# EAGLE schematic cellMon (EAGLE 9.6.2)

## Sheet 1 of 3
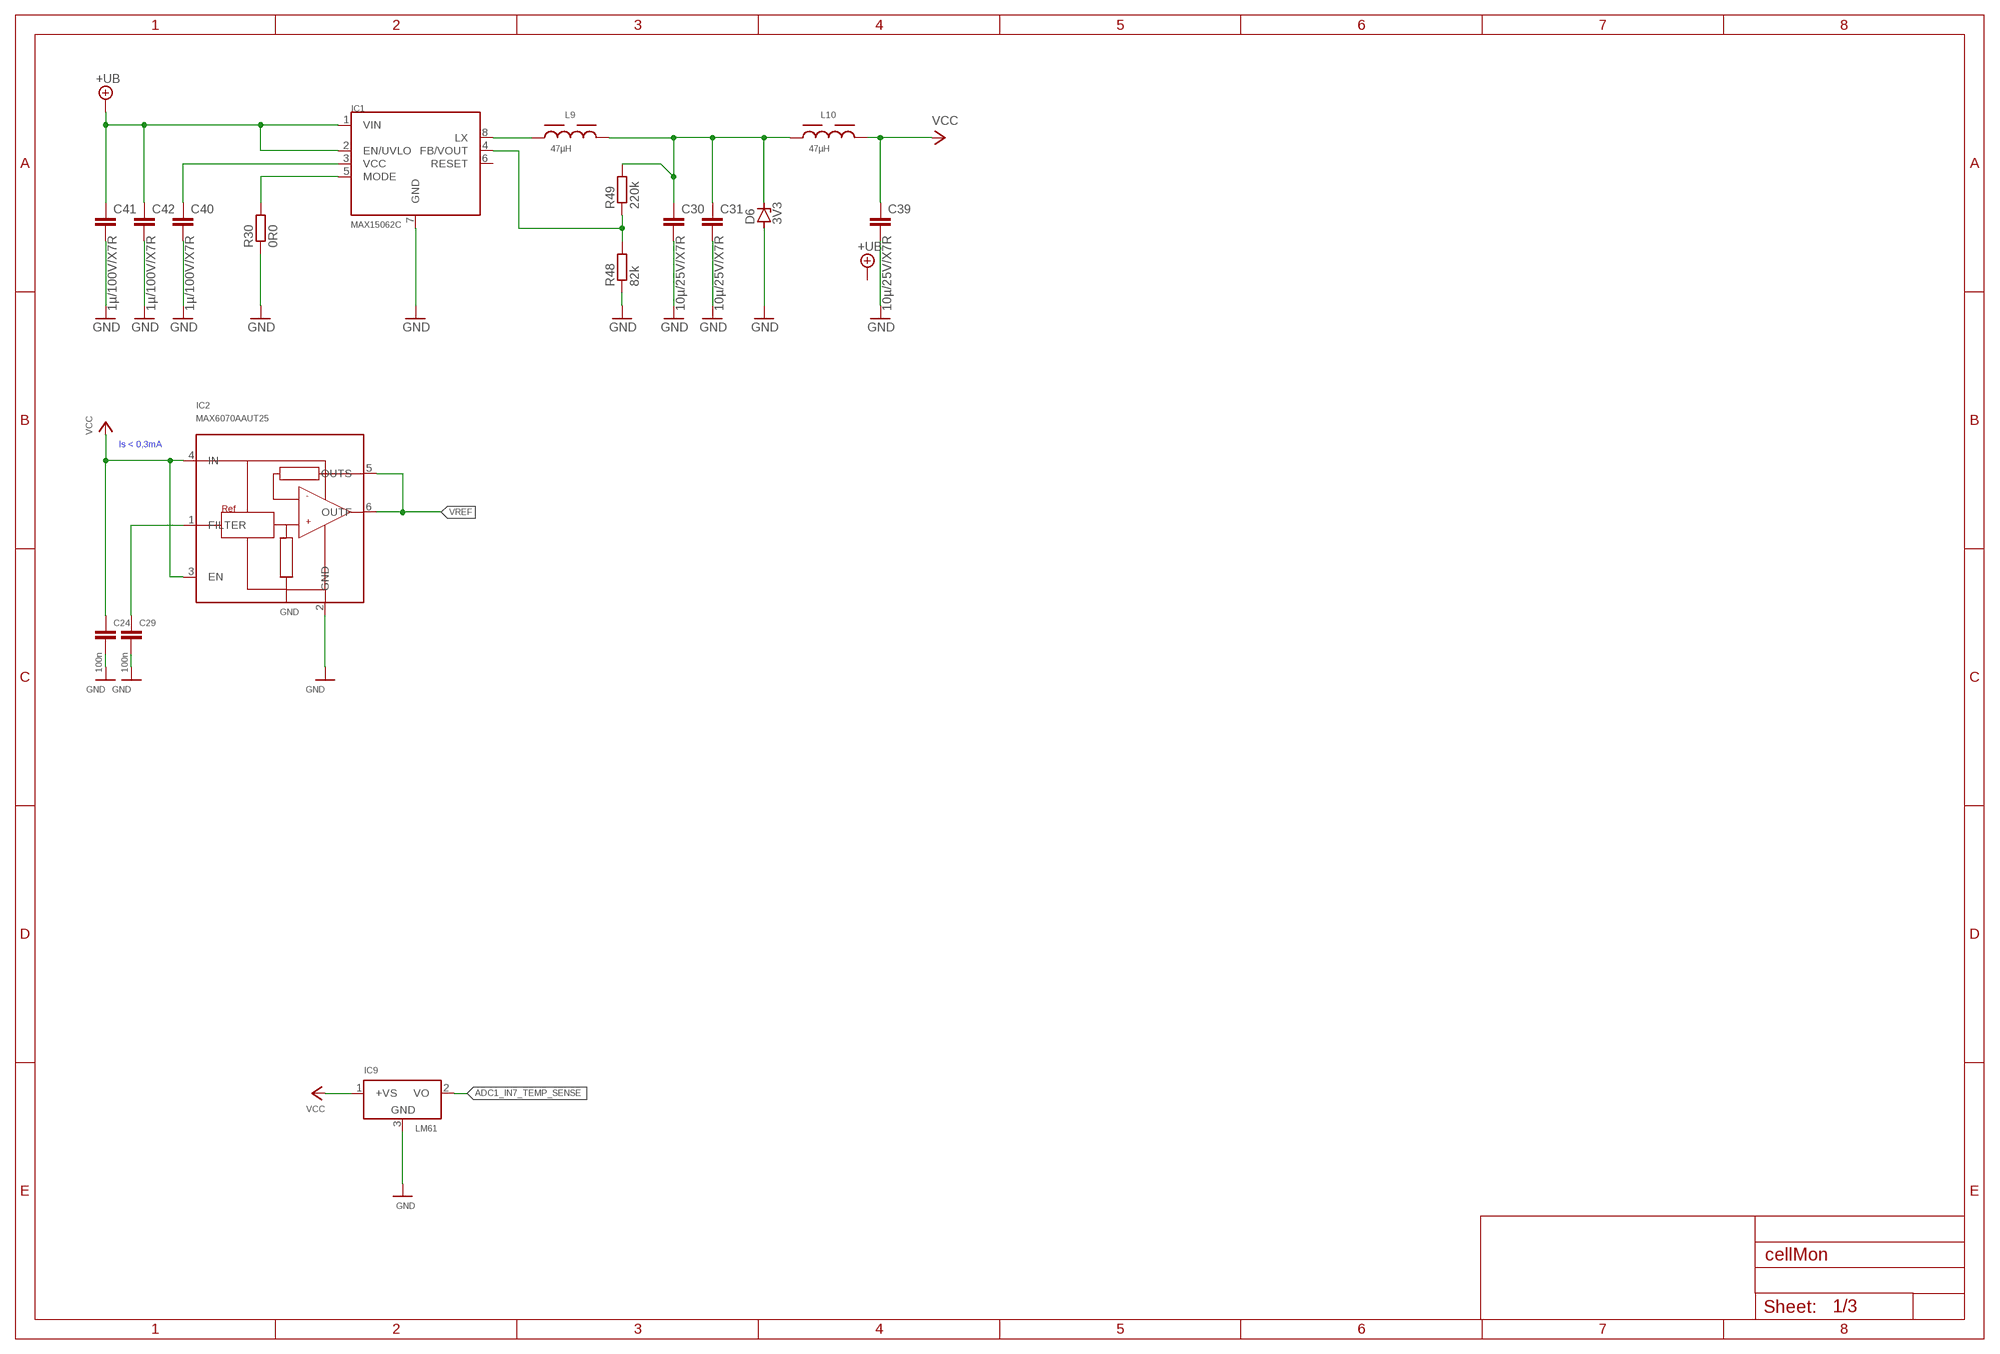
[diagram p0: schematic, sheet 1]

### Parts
C24  100n  C-EUC0603K  [C0603K]
C29  100n  C-EUC0603K  [C0603K]
C30  10µ/25V/X7R  C-EUC1210  [C1210]
C31  10µ/25V/X7R  C-EUC1210  [C1210]
C39  10µ/25V/X7R  C-EUC1210  [C1210]
C40  1µ/100V/X7R  C-EUC1210  [C1210]
C41  1µ/100V/X7R  C-EUC1210  [C1210]
C42  1µ/100V/X7R  C-EUC1210  [C1210]
D6  3V3  ZENER-DIODESOD80C  [SOD80C]
IC1  MAX15062C  MAX15062A  [8TDFN]
IC2  MAX6070AAUT25  MAX6070  [SOT23-6]
IC9  LM61  LM50  [SOT23]
L9  47µH  WE-LQS_4018_74404042470  [WE-LQS_4018]
L10  47µH  WE-LQS_4018_74404042470  [WE-LQS_4018]
R30  0R0  R-EU_R0603  [R0603]
R48  82k  R-EU_R0603  [R0603]
R49  220k  R-EU_R0603  [R0603]

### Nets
+UB: C41.1 C42.1 IC1.1(VIN) IC1.2(EN/UVLO)
ADC1_IN7_TEMP_SENSE: IC9.2(VO)
GND: C24.2 C29.2 C30.2 C31.2 C39.2 C40.2 C41.2 C42.2 D6.A IC1.7(GND) IC2.2(GND) IC9.3(GND) R30.1 R48.1 ; also sheet 2,3
N$1: C40.1 IC1.3(VCC)
N$3: C30.1 C31.1 D6.C L9.2 L10.1 R49.2
N$4: IC1.5(MODE) R30.2
N$12: IC1.8(LX) L9.1
N$21: IC1.4(FB/VOUT) R48.2 R49.1
N$22: C29.1 IC2.1(FILTER)
VCC: C24.1 C39.1 IC2.3(EN) IC2.4(IN) IC9.1(+VS) L10.2 ; also sheet 3
VREF: IC2.5(OUTS) IC2.6(OUTF)
Unconnected: IC1.6(RESET)

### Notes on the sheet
- Is < 0,3mA

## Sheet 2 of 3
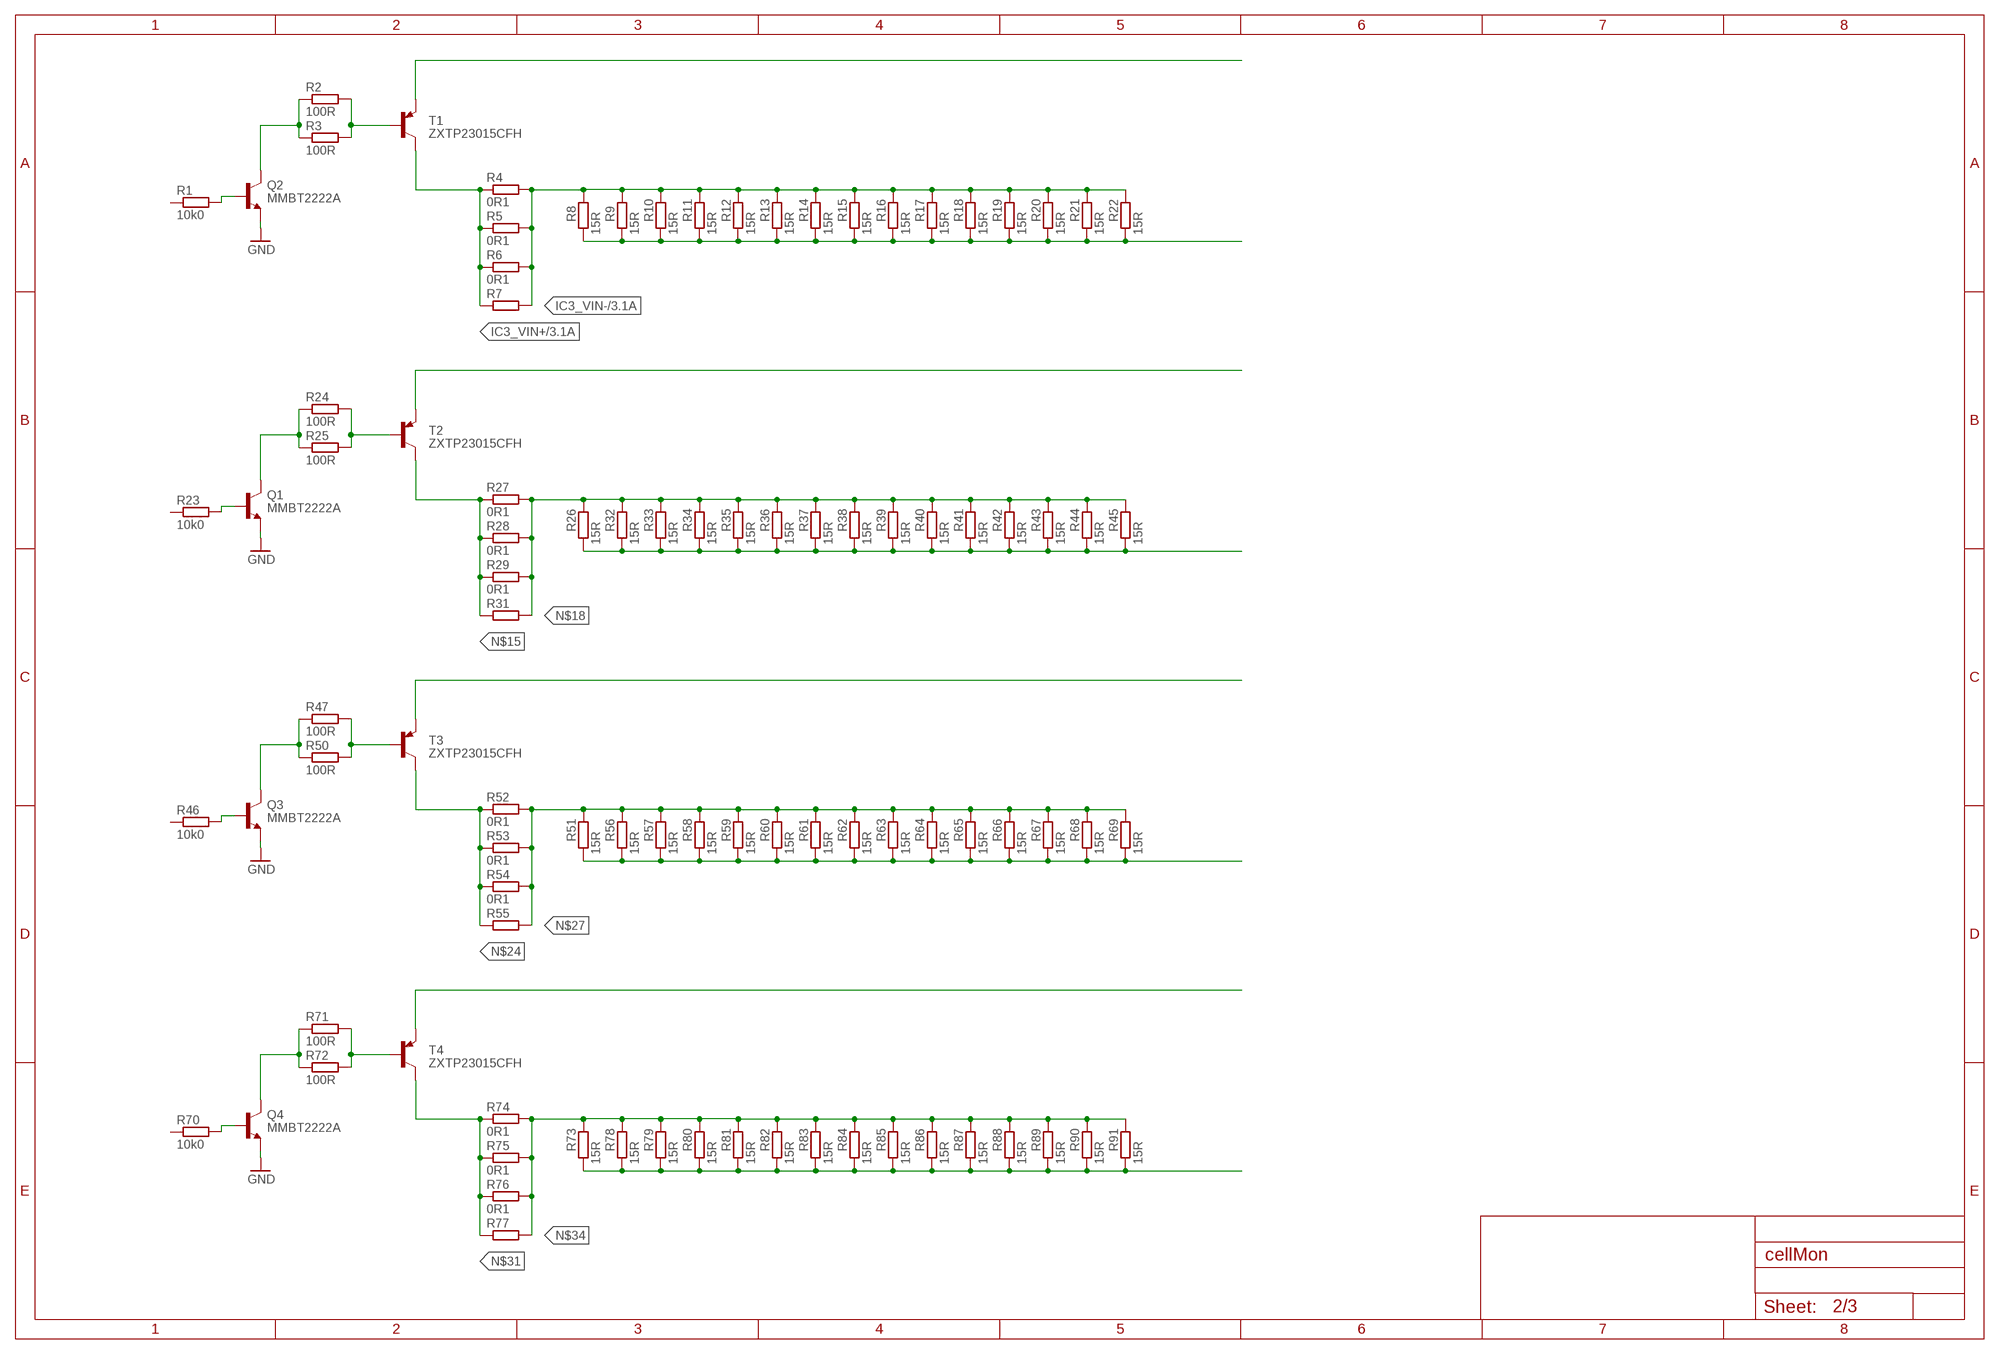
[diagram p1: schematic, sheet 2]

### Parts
Q1  MMBT2222A  BC817-40SMD  [SOT23-BEC]
Q2  MMBT2222A  BC817-40SMD  [SOT23-BEC]
Q3  MMBT2222A  BC817-40SMD  [SOT23-BEC]
Q4  MMBT2222A  BC817-40SMD  [SOT23-BEC]
R1  10k0  R-EU_R0603  [R0603]
R2  100R  R-EU_R0603  [R0603]
R3  100R  R-EU_R0603  [R0603]
R4  0R1  R-EU_R2010  [R2010]
R5  0R1  R-EU_R2010  [R2010]
R6  0R1  R-EU_R2010  [R2010]
R7  R-EU_R2010  [R2010]
R8  15R  R-EU_R2512  [R2512]
R9  15R  R-EU_R2512  [R2512]
R10  15R  R-EU_R2512  [R2512]
R11  15R  R-EU_R2512  [R2512]
R12  15R  R-EU_R2512  [R2512]
R13  15R  R-EU_R2512  [R2512]
R14  15R  R-EU_R2512  [R2512]
R15  15R  R-EU_R2512  [R2512]
R16  15R  R-EU_R2512  [R2512]
R17  15R  R-EU_R2512  [R2512]
R18  15R  R-EU_R2512  [R2512]
R19  15R  R-EU_R2512  [R2512]
R20  15R  R-EU_R2512  [R2512]
R21  15R  R-EU_R2512  [R2512]
R22  15R  R-EU_R2512  [R2512]
R23  10k0  R-EU_R0603  [R0603]
R24  100R  R-EU_R0603  [R0603]
R25  100R  R-EU_R0603  [R0603]
R26  15R  R-EU_R2512  [R2512]
R27  0R1  R-EU_R2010  [R2010]
R28  0R1  R-EU_R2010  [R2010]
R29  0R1  R-EU_R2010  [R2010]
R31  R-EU_R2010  [R2010]
R32  15R  R-EU_R2512  [R2512]
R33  15R  R-EU_R2512  [R2512]
R34  15R  R-EU_R2512  [R2512]
R35  15R  R-EU_R2512  [R2512]
R36  15R  R-EU_R2512  [R2512]
R37  15R  R-EU_R2512  [R2512]
R38  15R  R-EU_R2512  [R2512]
R39  15R  R-EU_R2512  [R2512]
R40  15R  R-EU_R2512  [R2512]
R41  15R  R-EU_R2512  [R2512]
R42  15R  R-EU_R2512  [R2512]
R43  15R  R-EU_R2512  [R2512]
R44  15R  R-EU_R2512  [R2512]
R45  15R  R-EU_R2512  [R2512]
R46  10k0  R-EU_R0603  [R0603]
R47  100R  R-EU_R0603  [R0603]
R50  100R  R-EU_R0603  [R0603]
R51  15R  R-EU_R2512  [R2512]
R52  0R1  R-EU_R2010  [R2010]
R53  0R1  R-EU_R2010  [R2010]
R54  0R1  R-EU_R2010  [R2010]
R55  R-EU_R2010  [R2010]
R56  15R  R-EU_R2512  [R2512]
R57  15R  R-EU_R2512  [R2512]
R58  15R  R-EU_R2512  [R2512]
R59  15R  R-EU_R2512  [R2512]
R60  15R  R-EU_R2512  [R2512]
R61  15R  R-EU_R2512  [R2512]
R62  15R  R-EU_R2512  [R2512]
R63  15R  R-EU_R2512  [R2512]
R64  15R  R-EU_R2512  [R2512]
R65  15R  R-EU_R2512  [R2512]
R66  15R  R-EU_R2512  [R2512]
R67  15R  R-EU_R2512  [R2512]
R68  15R  R-EU_R2512  [R2512]
R69  15R  R-EU_R2512  [R2512]
R70  10k0  R-EU_R0603  [R0603]
R71  100R  R-EU_R0603  [R0603]
R72  100R  R-EU_R0603  [R0603]
R73  15R  R-EU_R2512  [R2512]
R74  0R1  R-EU_R2010  [R2010]
R75  0R1  R-EU_R2010  [R2010]
R76  0R1  R-EU_R2010  [R2010]
R77  R-EU_R2010  [R2010]
R78  15R  R-EU_R2512  [R2512]
R79  15R  R-EU_R2512  [R2512]
R80  15R  R-EU_R2512  [R2512]
R81  15R  R-EU_R2512  [R2512]
R82  15R  R-EU_R2512  [R2512]
R83  15R  R-EU_R2512  [R2512]
R84  15R  R-EU_R2512  [R2512]
R85  15R  R-EU_R2512  [R2512]
R86  15R  R-EU_R2512  [R2512]
R87  15R  R-EU_R2512  [R2512]
R88  15R  R-EU_R2512  [R2512]
R89  15R  R-EU_R2512  [R2512]
R90  15R  R-EU_R2512  [R2512]
R91  15R  R-EU_R2512  [R2512]
T1  ZXTP23015CFH  BC807-16-PNP-SOT23-BEC  [SOT23-BEC]
T2  ZXTP23015CFH  BC807-16-PNP-SOT23-BEC  [SOT23-BEC]
T3  ZXTP23015CFH  BC807-16-PNP-SOT23-BEC  [SOT23-BEC]
T4  ZXTP23015CFH  BC807-16-PNP-SOT23-BEC  [SOT23-BEC]

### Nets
GND: Q1.E Q2.E Q3.E Q4.E ; also sheet 1,3
IC3_VIN+: R4.1 R5.1 R6.1 R7.1 T1.C ; also sheet 3
IC3_VIN-: R4.2 R5.2 R6.2 R7.2 R8.2 R9.2 R10.2 R11.2 R12.2 R13.2 R14.2 R15.2 R16.2 R17.2 R18.2 R19.2 R20.2 R21.2 R22.2 ; also sheet 3
N$2: Q2.C R2.1 R3.1
N$5: R2.2 R3.2 T1.B
N$6: Q1.C R24.1 R25.1
N$7: Q2.B R1.2
N$9: T1.E
N$10: R24.2 R25.2 T2.B
N$11: Q1.B R23.2
N$13: R8.1 R9.1 R10.1 R11.1 R12.1 R13.1 R14.1 R15.1 R16.1 R17.1 R18.1 R19.1 R20.1 R21.1 R22.1
N$15: R27.1 R28.1 R29.1 R31.1 T2.C
N$16: T2.E
N$17: R26.1 R32.1 R33.1 R34.1 R35.1 R36.1 R37.1 R38.1 R39.1 R40.1 R41.1 R42.1 R43.1 R44.1 R45.1
N$18: R26.2 R27.2 R28.2 R29.2 R31.2 R32.2 R33.2 R34.2 R35.2 R36.2 R37.2 R38.2 R39.2 R40.2 R41.2 R42.2 R43.2 R44.2 R45.2
N$19: Q3.C R47.1 R50.1
N$20: R47.2 R50.2 T3.B
N$23: Q3.B R46.2
N$24: R52.1 R53.1 R54.1 R55.1 T3.C
N$25: T3.E
N$26: R51.1 R56.1 R57.1 R58.1 R59.1 R60.1 R61.1 R62.1 R63.1 R64.1 R65.1 R66.1 R67.1 R68.1 R69.1
N$27: R51.2 R52.2 R53.2 R54.2 R55.2 R56.2 R57.2 R58.2 R59.2 R60.2 R61.2 R62.2 R63.2 R64.2 R65.2 R66.2 R67.2 R68.2 R69.2
N$28: Q4.C R71.1 R72.1
N$29: R71.2 R72.2 T4.B
N$30: Q4.B R70.2
N$31: R74.1 R75.1 R76.1 R77.1 T4.C
N$32: T4.E
N$33: R73.1 R78.1 R79.1 R80.1 R81.1 R82.1 R83.1 R84.1 R85.1 R86.1 R87.1 R88.1 R89.1 R90.1 R91.1
N$34: R73.2 R74.2 R75.2 R76.2 R77.2 R78.2 R79.2 R80.2 R81.2 R82.2 R83.2 R84.2 R85.2 R86.2 R87.2 R88.2 R89.2 R90.2 R91.2
Unconnected: R1.1 R23.1 R46.1 R70.1

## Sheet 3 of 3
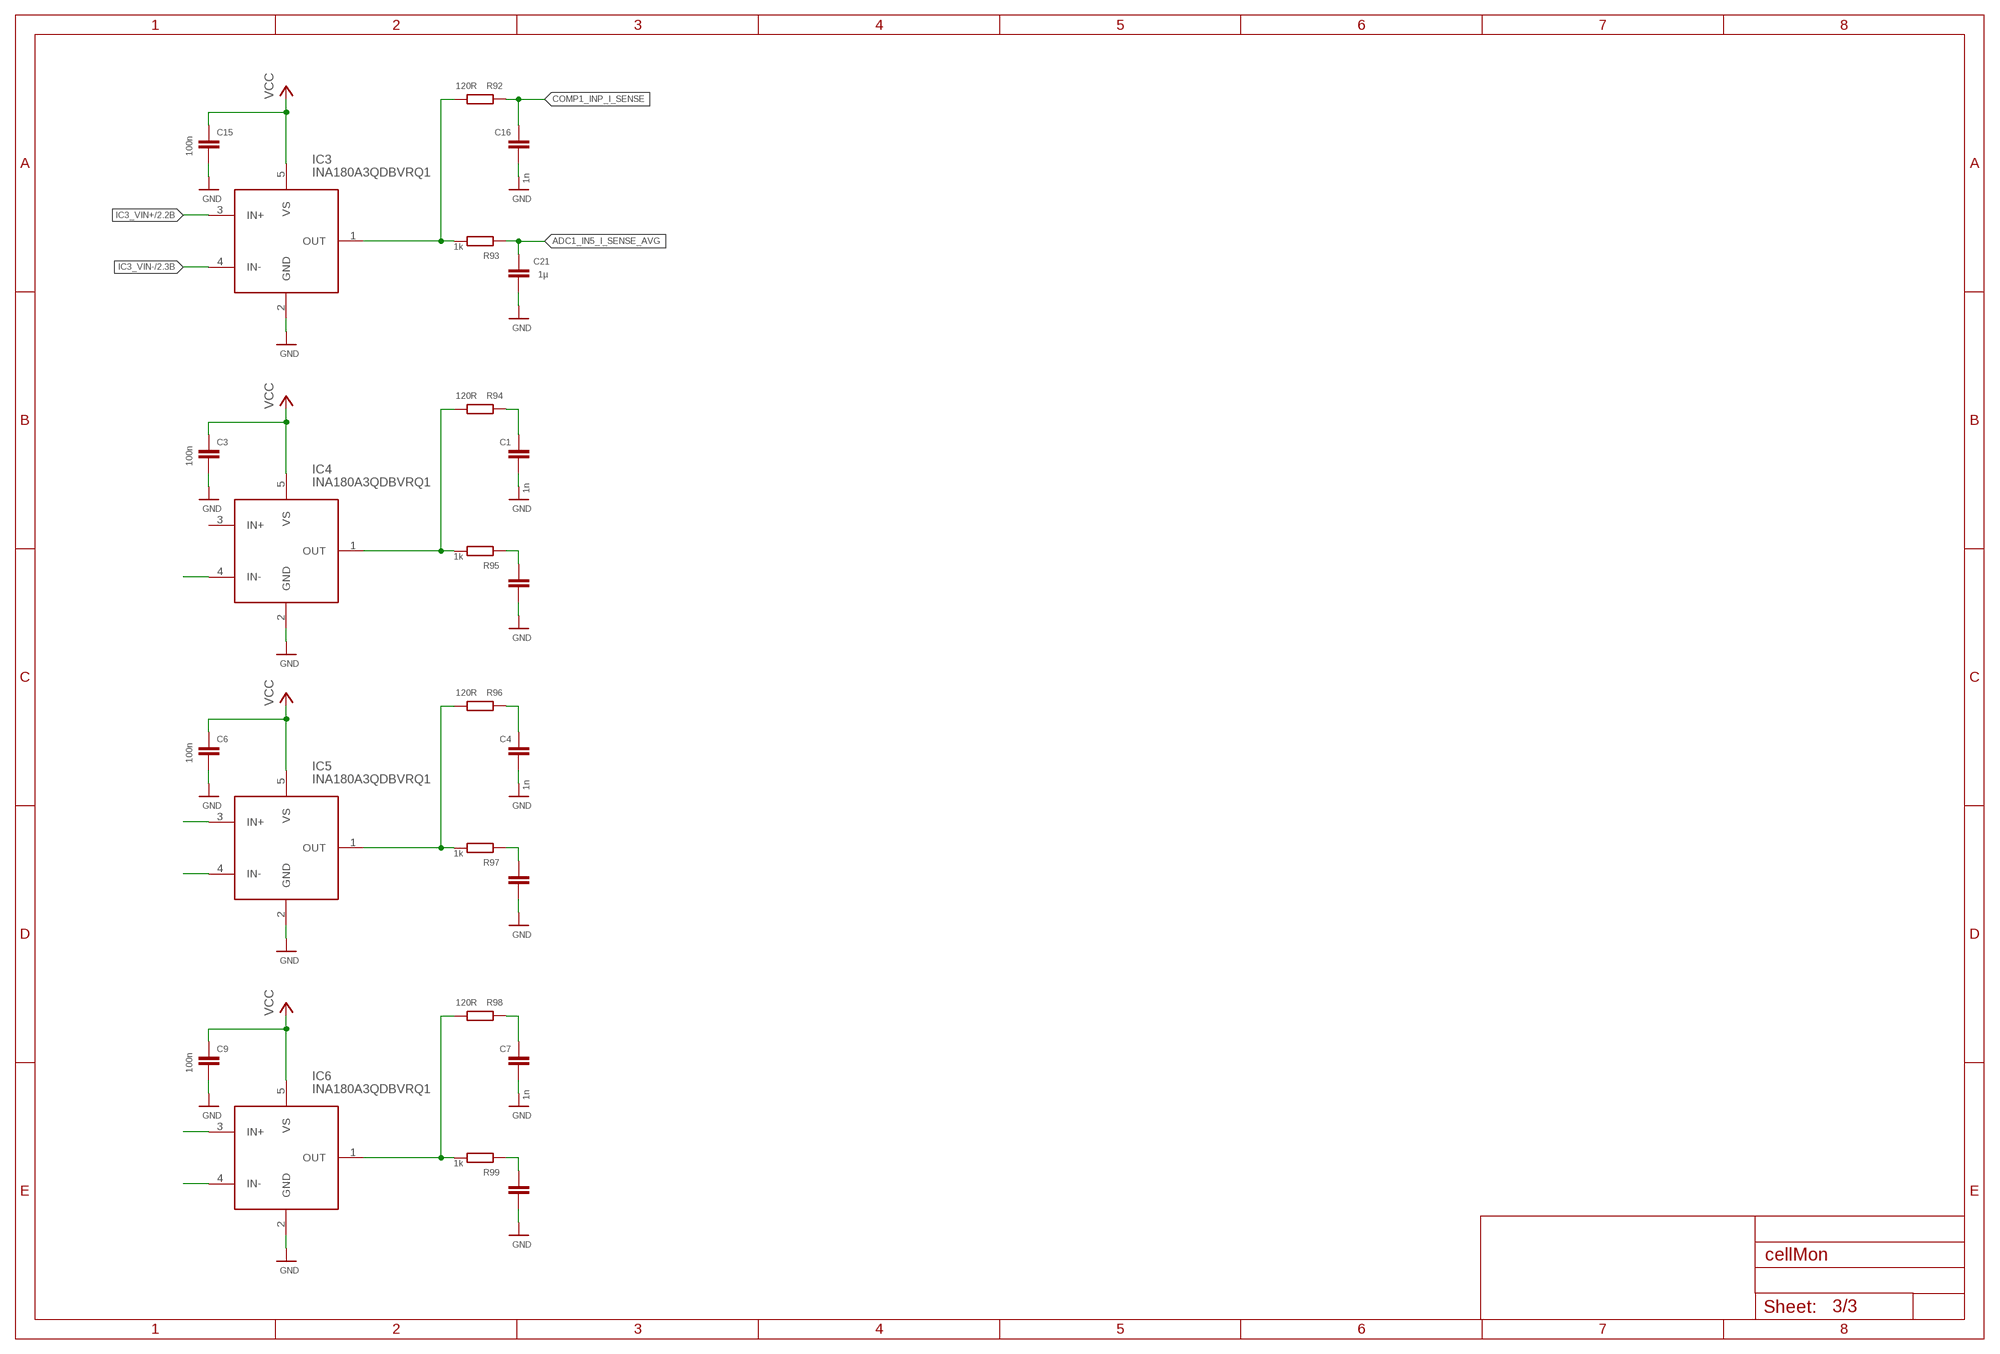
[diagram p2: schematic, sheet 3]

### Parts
C1  1n  C-EUC0603  [C0603]
C2  1µ  C-EUC0603  [C0603]
C3  100n  C-EUC0603K  [C0603K]
C4  1n  C-EUC0603  [C0603]
C5  1µ  C-EUC0603  [C0603]
C6  100n  C-EUC0603K  [C0603K]
C7  1n  C-EUC0603  [C0603]
C8  1µ  C-EUC0603  [C0603]
C9  100n  C-EUC0603K  [C0603K]
C15  100n  C-EUC0603K  [C0603K]
C16  1n  C-EUC0603  [C0603]
C21  1µ  C-EUC0603  [C0603]
IC3  INA180A3QDBVRQ1  INA180A  [SOT95P280X110-5N]
IC4  INA180A3QDBVRQ1  INA180A  [SOT95P280X110-5N]
IC5  INA180A3QDBVRQ1  INA180A  [SOT95P280X110-5N]
IC6  INA180A3QDBVRQ1  INA180A  [SOT95P280X110-5N]
R92  120R  R-EU_R0603  [R0603]
R93  1k  R-EU_R0603  [R0603]
R94  120R  R-EU_R0603  [R0603]
R95  1k  R-EU_R0603  [R0603]
R96  120R  R-EU_R0603  [R0603]
R97  1k  R-EU_R0603  [R0603]
R98  120R  R-EU_R0603  [R0603]
R99  1k  R-EU_R0603  [R0603]

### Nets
ADC1_IN5_I_SENSE_AVG: C2.1 C5.1 C8.1 C21.1 R93.1 R95.1 R97.1 R99.1
COMP1_INP_I_SENSE: C1.1 C4.1 C7.1 C16.1 R92.1 R94.1 R96.1 R98.1
GND: C1.2 C2.2 C3.2 C4.2 C5.2 C6.2 C7.2 C8.2 C9.2 C15.2 C16.2 C21.2 IC3.2(GND) IC4.2(GND) IC5.2(GND) IC6.2(GND) ; also sheet 1,2
IC1_VIN+: IC5.3(IN+) IC6.3(IN+)
IC3_VIN+: IC3.3(IN+) ; also sheet 2
IC3_VIN-: IC3.4(IN-) IC4.4(IN-) IC5.4(IN-) IC6.4(IN-) ; also sheet 2
N$8: IC4.1(OUT) R94.2 R95.2
N$14: IC5.1(OUT) R96.2 R97.2
N$35: IC3.1(OUT) R92.2 R93.2
N$36: IC6.1(OUT) R98.2 R99.2
VCC: C3.1 C6.1 C9.1 C15.1 IC3.5(VS) IC4.5(VS) IC5.5(VS) IC6.5(VS) ; also sheet 1
Unconnected: IC4.3(IN+)

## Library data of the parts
C1 C4 C7 C16 = rcl:C-EU: CAPACITOR, European symbol; PARTNO: C043; SPICEPREFIX: C
C2 C5 C8 C21 = rcl:C-EU: CAPACITOR, European symbol; PARTNO: C079; SPICEPREFIX: C
C3 C6 C9 C15 C24 C29 = rcl:C-EU: CAPACITOR, European symbol; PARTNO: C067; SPICEPREFIX: C
C30 C31 C39 = rcl:C-EU: CAPACITOR, European symbol; PARTNO: C218; SPICEPREFIX: C
C40-C42 = rcl:C-EU: CAPACITOR, European symbol; PARTNO: C216; SPICEPREFIX: C
D6 = diode:ZENER-DIODE: Z-Diode; PARTNO: D007
IC1 = MAX15062A:MAX15062A: 60V, 300mA, Ultra-Small, High-Efficiency, Synchronous Step-Down DC-DC Converters; PARTNO: IC292
IC2 = max6070:MAX6070; PARTNO: IC326
IC3-IC6 = ina180:INA180: Unidrectional current Sense Verstärkung 20/50/100/200; PARTNO: IC325
IC9 = linear:LM50: SOT-23 Single-Supply Centigrade Temperature Sensor Vout = (10mV/°C x Temp °C) +5mmmV Source: http://cache.national.com/ds/LM/LM50.pdf; PARTNO: IC040
L9 L10 = Wurth_Power Magnetics_WE-LQS:WE-LQS_4018: WE-LQS SMD Power Inductor; DATASHEET-URL: https://www.we-online.com/catalog/datasheet/74404042470.pdf; FRES: 11MHz; IR: 0.6A; ISAT: 0.7A; PART-NUMBER: 74404042470; PARTNO: L122; RDC: 620mOhm; VALUE: 47uH
Q1-Q4 = transistor-npn:BC817*: NPN Transistor; PARTNO: T066
R1 R23 R46 R70 = rcl:R-EU_: RESISTOR, European symbol; PARTNO: R221; SPICEPREFIX: R
R2 R3 R24 R25 R47 R50 R71 R72 = rcl:R-EU_: RESISTOR, European symbol; PARTNO: R173; SPICEPREFIX: R
R4-R7 R27-R29 R31 R52-R55 R74-R77 = rcl:R-EU_: RESISTOR, European symbol; PARTNO: R496; SPICEPREFIX: R
R8-R22 R26 R32-R45 R51 R56-R69 R73 R78-R91 = rcl:R-EU_: RESISTOR, European symbol; PARTNO: R500; SPICEPREFIX: R
R30 = rcl:R-EU_: RESISTOR, European symbol; PARTNO: R504; SPICEPREFIX: R
R48 = rcl:R-EU_: RESISTOR, European symbol; PARTNO: R243; SPICEPREFIX: R
R49 = rcl:R-EU_: RESISTOR, European symbol; PARTNO: R253; SPICEPREFIX: R
R92 R94 R96 R98 = rcl:R-EU_: RESISTOR, European symbol; PARTNO: R175; SPICEPREFIX: R
R93 R95 R97 R99 = rcl:R-EU_: RESISTOR, European symbol; PARTNO: R197; SPICEPREFIX: R
T1-T4 = transistor:*-PNP-: PNP Transistror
